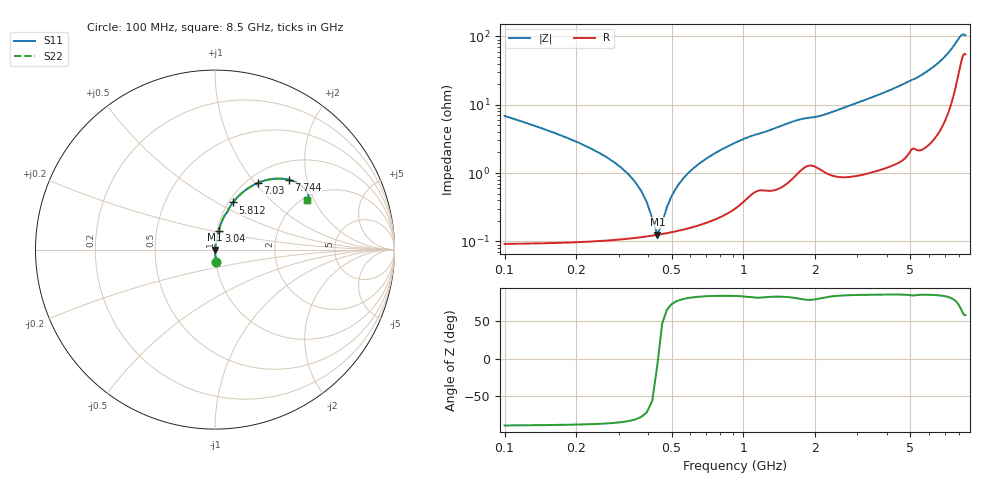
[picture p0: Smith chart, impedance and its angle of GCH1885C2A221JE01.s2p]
!Murata Part Number: GCH1885C2A221JE01
!These Parameters are Measured in Series Mode Connection
!Data Generated on Jun 19, 2026
!  o--ll--o
!Port1  Port2
!  o------o
!Operation Temp=25[degC], DC Bias Voltage=0[V]
!Freq. Start=100[MHz] Stop=9[GHz] 401[Steps]
# Hz S RI R 50
!Freq.(Hz) S11(Real) S11(Imag) S21(Real) S21(Imag) S12(Real) S12(Imag) S22(Real) S22(Imag)
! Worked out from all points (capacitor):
!   401 points, 100 MHz to 8.5 GHz, reference 50 ohm
!   read as one part in series: C = 220 pF near 142 MHz
!   lowest |Z| = 126 mohm at 436 MHz (marker M1)
!   series resonance near 438.5 MHz, so ESL is about 600 pH
!   S11 on the Smith chart (normalised r, x): 100 MHz: 1.00, -0.14; 3.04 GHz: 1.02, +0.22; 5.812 GHz: 1.05, +0.60; 7.03 GHz: 1.12, +1.03; 7.744 GHz: 1.37, +1.56; 8.5 GHz: 2.09, +1.77
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1e8  0.00559 -0.0681  0.9944 0.0681  0.9944 0.0681  0.00559 -0.0681
3.1e8  0.00121 -0.0117  0.9988 0.0117  0.9988 0.0117  0.00121 -0.0117
3.52e8  0.00117 -0.00731  0.9988 0.00731  0.9988 0.00731  0.00117 -0.00731
4.15e8  0.00121 -0.00182  0.9988 0.00182  0.9988 0.00182  0.00121 -0.00182
4.36e8  0.00124 -0.000189  0.9988 0.000189  0.9988 0.000189  0.00124 -0.000189
4.78e8  0.00133 0.00286  0.9987 -0.00286  0.9987 -0.00286  0.00133 0.00286
5.2e8  0.00143 0.00567  0.9986 -0.00567  0.9986 -0.00567  0.00143 0.00567
5.62e8  0.00156 0.00831  0.9984 -0.00831  0.9984 -0.00831  0.00156 0.00831
6.25e8  0.00179 0.012  0.9982 -0.012  0.9982 -0.012  0.00179 0.012
7.3e8  0.00228 0.0177  0.9977 -0.0177  0.9977 -0.0177  0.00228 0.0177
1.024e9  0.00508 0.032  0.9949 -0.032  0.9949 -0.032  0.00508 0.032
1.507e9  0.0094 0.0509  0.9906 -0.0509  0.9906 -0.0509  0.0094 0.0509
2.914e9  0.019 0.0996  0.981 -0.0996  0.981 -0.0996  0.019 0.0996
3.04e9  0.0204 0.1051  0.9796 -0.1051  0.9796 -0.1051  0.0204 0.1051
4.3e9  0.0417 0.1655  0.9583 -0.1655  0.9583 -0.1655  0.0417 0.1655
5.707e9  0.0936 0.2542  0.9064 -0.2542  0.9064 -0.2542  0.0936 0.2542
5.812e9  0.1001 0.2629  0.8999 -0.2629  0.8999 -0.2629  0.1001 0.2629
7.03e9  0.2384 0.371  0.7616 -0.371  0.7616 -0.371  0.2384 0.371
7.114e9  0.2545 0.3774  0.7455 -0.3774  0.7455 -0.3774  0.2545 0.3774
7.744e9  0.4114 0.3886  0.5886 -0.3886  0.5886 -0.3886  0.4114 0.3886
8.164e9  0.5111 0.3224  0.4889 -0.3224  0.4889 -0.3224  0.5111 0.3224
8.5e9  0.5125 0.2782  0.4875 -0.2782  0.4875 -0.2782  0.5125 0.2782
